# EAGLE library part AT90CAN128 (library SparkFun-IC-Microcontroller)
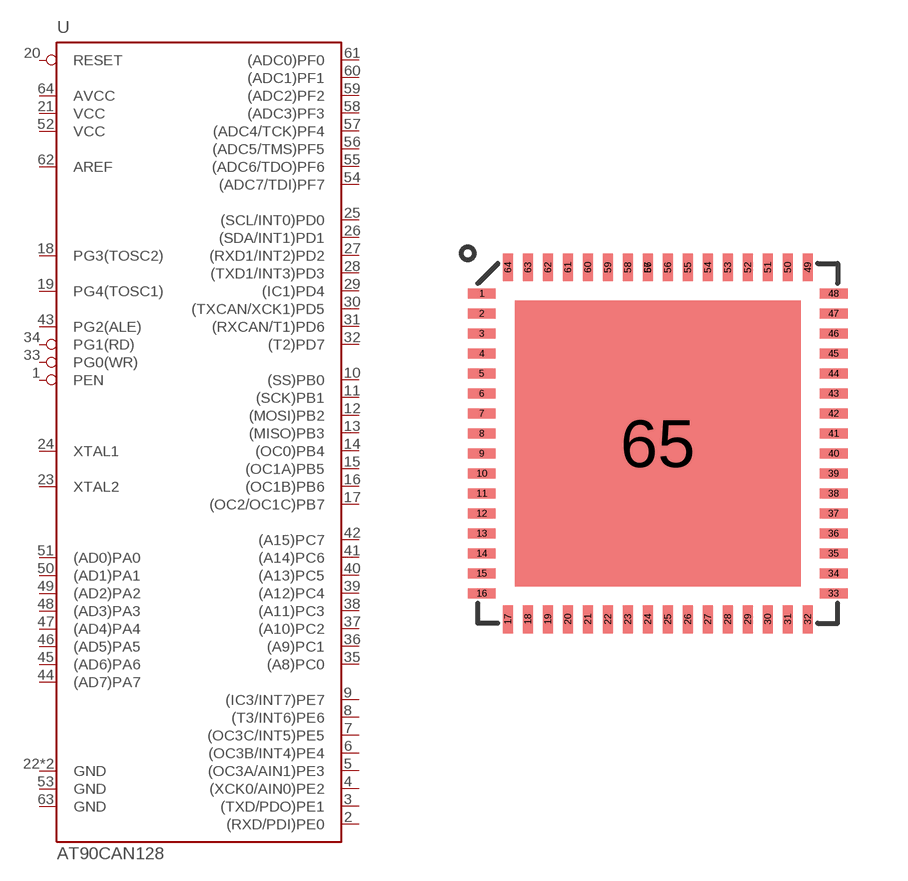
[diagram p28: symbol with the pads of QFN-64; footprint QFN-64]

Designator prefix U

## AT90CAN128 (PROD_ID: IC-13822)  [QFN-64]
1  PEN
2  (RXD/PDI)PE0
3  (TXD/PDO)PE1
4  (XCK0/AIN0)PE2
5  (OC3A/AIN1)PE3
6  (OC3B/INT4)PE4
7  (OC3C/INT5)PE5
8  (T3/INT6)PE6
9  (IC3/INT7)PE7
10  (SS)PB0
11  (SCK)PB1
12  (MOSI)PB2
13  (MISO)PB3
14  (OC0)PB4
15  (OC1A)PB5
16  (OC1B)PB6
17  (OC2/OC1C)PB7
18  PG3(TOSC2)
19  PG4(TOSC1)
20  RESET
21  VCC
22  GND
23  XTAL2
24  XTAL1
25  (SCL/INT0)PD0
26  (SDA/INT1)PD1
27  (RXD1/INT2)PD2
28  (TXD1/INT3)PD3
29  (IC1)PD4
30  (TXCAN/XCK1)PD5
31  (RXCAN/T1)PD6
32  (T2)PD7
33  PG0(WR)
34  PG1(RD)
35  (A8)PC0
36  (A9)PC1
37  (A10)PC2
38  (A11)PC3
39  (A12)PC4
40  (A13)PC5
41  (A14)PC6
42  (A15)PC7
43  PG2(ALE)
44  (AD7)PA7
45  (AD6)PA6
46  (AD5)PA5
47  (AD4)PA4
48  (AD3)PA3
49  (AD2)PA2
50  (AD1)PA1
51  (AD0)PA0
52  VCC
53  GND
54  (ADC7/TDI)PF7
55  (ADC6/TDO)PF6
56  (ADC5/TMS)PF5
57  (ADC4/TCK)PF4
58  (ADC3)PF3
59  (ADC2)PF2
60  (ADC1)PF1
61  (ADC0)PF0
62  AREF
63  GND
64  AVCC
65  GND

## Footprint QFN-64 (pad centres in mm)
smd 0.7 x 0.25: 1 -4.4,3.75; 2 -4.4,3.25; 3 -4.4,2.75; 4 -4.4,2.25; 5 -4.4,1.75; 6 -4.4,1.25; 7 -4.4,0.75; 8 -4.4,0.25; 9 -4.4,-0.25; 10 -4.4,-0.75; 11 -4.4,-1.25; 12 -4.4,-1.75; 13 -4.4,-2.25; 14 -4.4,-2.75; 15 -4.4,-3.25; 16 -4.4,-3.75; 33 4.4,-3.75; 34 4.4,-3.25; 35 4.4,-2.75; 36 4.4,-2.25; 37 4.4,-1.75; 38 4.4,-1.25; 39 4.4,-0.75; 40 4.4,-0.25; 41 4.4,0.25; 42 4.4,0.75; 43 4.4,1.25; 44 4.4,1.75; 45 4.4,2.25; 46 4.4,2.75; 47 4.4,3.25; 48 4.4,3.75
smd 0.25 x 0.7: 17 -3.75,-4.4; 18 -3.25,-4.4; 19 -2.75,-4.4; 20 -2.25,-4.4; 21 -1.75,-4.4; 22 -1.25,-4.4; 23 -0.75,-4.4; 24 -0.25,-4.4; 25 0.25,-4.4; 26 0.75,-4.4; 27 1.25,-4.4; 28 1.75,-4.4; 29 2.25,-4.4; 30 2.75,-4.4; 31 3.25,-4.4; 32 3.75,-4.4; 49 3.75,4.4; 50 3.25,4.4; 51 2.75,4.4; 52 2.25,4.4; 53 1.75,4.4; 54 1.25,4.4; 55 0.75,4.4; 56 0.25,4.4; 57 -0.25,4.4; 58 -0.75,4.4; 59 -1.25,4.4; 60 -1.75,4.4; 61 -2.25,4.4; 62 -2.75,4.4; 63 -3.25,4.4; 64 -3.75,4.4; 66 -0.25,4.4
smd 7.15 x 7.15: 65 0,0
